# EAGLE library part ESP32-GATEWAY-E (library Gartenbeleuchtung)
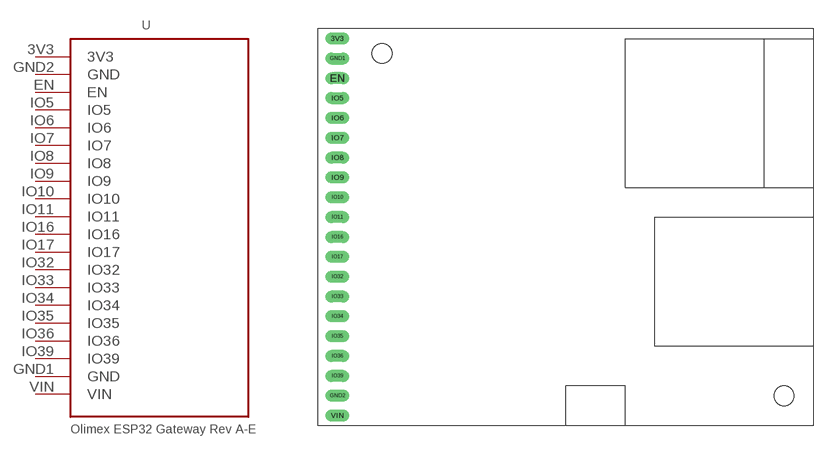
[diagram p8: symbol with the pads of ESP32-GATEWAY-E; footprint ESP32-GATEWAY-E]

Designator prefix -

## ESP32-GATEWAY-E  [ESP32-GATEWAY-E]
3V3  3V3  pwr
EN  EN
GND1  GND  pwr
GND2  GND  pwr
IO5  IO5
IO6  IO6
IO7  IO7
IO8  IO8
IO9  IO9
IO10  IO10
IO11  IO11
IO16  IO16
IO17  IO17
IO32  IO32
IO33  IO33
IO34  IO34
IO35  IO35
IO36  IO36
IO39  IO39
VIN  VIN  pwr

## Footprint ESP32-GATEWAY-E (pad centres in mm)
drill 1 pad 1.422 long: 3V3 0,0; EN 0,-5.08; GND1 0,-2.54; GND2 0,-45.72; IO5 0,-7.62; IO6 0,-10.16; IO7 0,-12.7; IO8 0,-15.24; IO9 0,-17.78; IO10 0,-20.32; IO11 0,-22.86; IO16 0,-25.4; IO17 0,-27.94; IO32 0,-30.48; IO33 0,-33.02; IO34 0,-35.56; IO35 0,-38.1; IO36 0,-40.64; IO39 0,-43.18; VIN 0,-48.26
